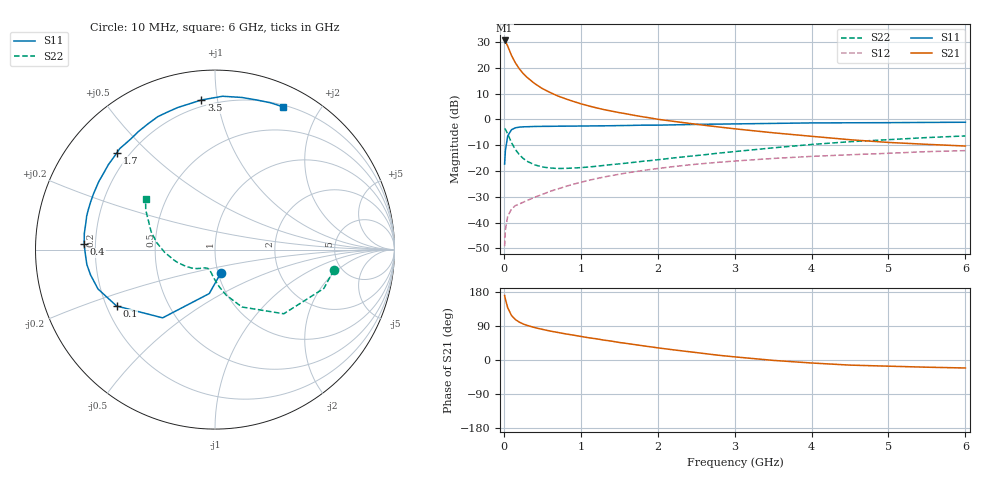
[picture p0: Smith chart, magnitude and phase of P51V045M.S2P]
! SIEMENS Small Signal Semiconductors
! BFP183
! Si NPN RF Bipolar Junction Transistor in SOT143
! VCE = 1 V  IC = 45 mA
! Common Emitter S-Parameters:  March  1996
# GHz  S  MA  R  50
!  f  S11  S21  S12  S22
! GHz  MAG  ANG  MAG  ANG  MAG  ANG  MAG  ANG
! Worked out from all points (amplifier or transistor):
!   36 points, 10 MHz to 6 GHz, reference 50 ohm
!   highest |S21| = 30.6 dB at 10 MHz (marker M1)
!   |S21| within 3 dB of that: start of sweep to 61.14 MHz
!   unconditionally stable (mu >= 1): start of sweep to 26.6 MHz; 179.8 MHz to end of sweep
!   at 250 MHz: K = 1.21, MAG = 22.2 dB, |S12| = -32.1 dB
!   at 1.4 GHz: K = 1.85, MAG = 7.2 dB, |S12| = -21.8 dB
!   at 6 GHz: K = 1.49, MAG = -3.3 dB, |S12| = -12.1 dB
!   S11 on the Smith chart (normalised r, x): 10 MHz: 1.03, -0.28; 100 MHz: 0.24, -0.25; 400 MHz: 0.16, +0.02; 1.7 GHz: 0.15, +0.40; 3.5 GHz: 0.16, +0.90; 6 GHz: 0.22, +1.56
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0.01  0.1366 -76.9  33.87 170.2  0.0035 66.2  0.6719 -9.7
0.02  0.2469 -97.4  32.76 160.9  0.0072 68.4  0.6441 -19.6
0.05  0.4793 -127.5  26.34 138.0  0.0133 54.8  0.5242 -43.0
0.1  0.6321 -150.2  17.29 117.3  0.0184 42.8  0.3531 -64.9
0.15  0.6878 -161.4  12.49 106.7  0.0214 40.8  0.2606 -76.3
0.2  0.7076 -168.5  9.628 100.0  0.0229 42.2  0.2087 -83.4
0.25  0.7187 -173.3  7.796 95.2  0.0248 44.0  0.1762 -88.8
0.3  0.7215 -176.9  6.557 91.5  0.0267 46.5  0.1551 -93.1
0.4  0.73 177.6  4.962 85.6  0.031 50.8  0.1319 -98.9
0.5  0.7336 172.9  3.962 80.9  0.0352 52.7  0.1199 -103.7
0.6  0.7345 168.7  3.331 76.5  0.0404 55.1  0.1146 -107.9
0.7  0.739 165.3  2.852 72.8  0.0449 56.9  0.112 -111.2
0.9  0.7422 158.9  2.245 65.8  0.0554 57.7  0.1143 -116.0
1.1  0.7467 152.4  1.832 58.8  0.0659 57.9  0.1196 -121.2
1.3  0.7516 146.5  1.551 52.5  0.0765 57.1  0.1284 -125.8
1.7  0.7682 135.3  1.196 40.7  0.0968 54.3  0.1479 -134.5
2.2  0.7843 122.8  0.919 26.9  0.1216 49.1  0.1788 -147.2
2.8  0.8113 108.7  0.712 12.3  0.1481 42.1  0.2228 -161.7
3.5  0.8369 95.2  0.551 -1.0  0.1752 34.4  0.2814 -177.0
4.5  0.8607 80.0  0.404 -13.5  0.2066 23.2  0.3701 164.2
5.5  0.8746 69.2  0.329 -19.0  0.2373 13.5  0.4447 150.2
6  0.8813 64.5  0.305 -21.1  0.2485 8.3  0.4787 143.9
